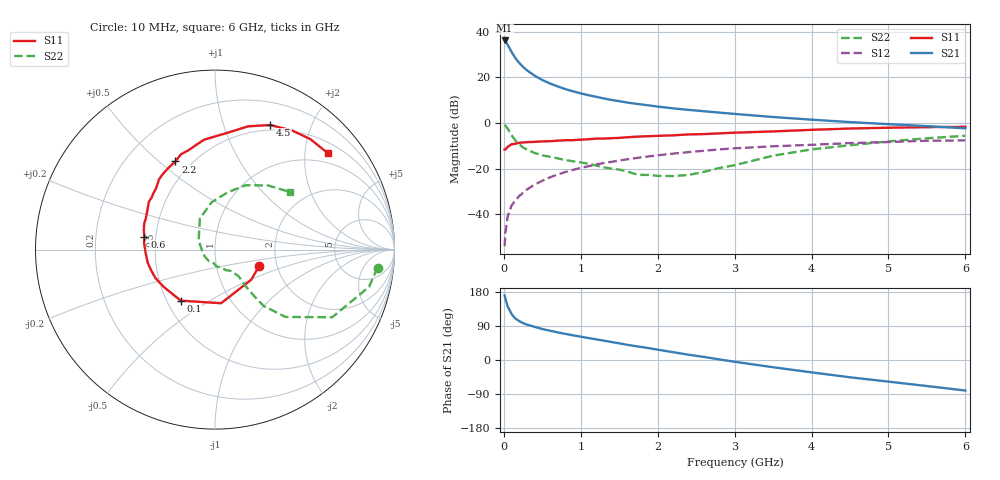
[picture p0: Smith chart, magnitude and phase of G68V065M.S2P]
! SIEMENS Small Signal Semiconductors
! BFG193
! Si NPN RF Bipolar Junction Transistor in SOT223
! VCE = 8 V  IC = 65 mA
! Common Emitter S-Parameters:  August  1996
# GHz  S  MA  R  50
!  f  S11  S21  S12  S22
! GHz  MAG  ANG  MAG  ANG  MAG  ANG  MAG  ANG
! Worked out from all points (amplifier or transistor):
!   36 points, 10 MHz to 6 GHz, reference 50 ohm
!   highest |S21| = 36.2 dB at 10 MHz (marker M1)
!   |S21| within 3 dB of that: start of sweep to 67.71 MHz
!   unconditionally stable (mu >= 1): 431.1 MHz to 2.36 GHz
!   at 250 MHz: K = 0.93, MSG = 27.6 dB, |S12| = -30.5 dB
!   at 1.4 GHz: K = 1.05, MAG = 12.3 dB, |S12| = -17.0 dB
!   at 6 GHz: K = 0.89, MSG = 2.7 dB, |S12| = -7.6 dB
!   S11 on the Smith chart (normalised r, x): 10 MHz: 1.62, -0.31; 100 MHz: 0.59, -0.38; 600 MHz: 0.43, +0.07; 2.2 GHz: 0.41, +0.57; 4.5 GHz: 0.44, +1.44; 6 GHz: 0.74, +2.51
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0.01  0.2628 -20.0  64.75 170.4  0.002 84.1  0.9112 -6.3
0.02  0.2626 -39.7  62.49 162.6  0.0039 74.0  0.8829 -13.6
0.05  0.3007 -83.5  52.02 141.3  0.0091 69.7  0.754 -30.0
0.1  0.3424 -123.8  36.41 121.5  0.0155 66.1  0.5431 -43.7
0.15  0.3532 -143.8  26.54 109.3  0.0202 66.5  0.4148 -49.2
0.2  0.3682 -154.6  20.88 102.6  0.025 67.8  0.3433 -49.8
0.25  0.3749 -162.9  17.02 97.3  0.0297 68.6  0.2919 -50.0
0.3  0.3818 -168.9  14.37 93.4  0.035 70.0  0.2631 -50.0
0.4  0.3871 -177.4  10.95 87.5  0.0447 69.6  0.2207 -49.1
0.5  0.3968 174.7  8.789 81.8  0.0544 68.9  0.1962 -48.5
0.6  0.4002 169.5  7.379 77.3  0.0646 68.0  0.1818 -49.5
0.7  0.4114 164.6  6.357 72.9  0.0747 66.8  0.1683 -51.4
0.8  0.4205 159.7  5.554 68.9  0.0845 64.6  0.1544 -53.0
1.1  0.4424 147.7  4.082 58.0  0.1131 59.6  0.1281 -62.8
1.3  0.4566 140.8  3.466 51.0  0.1331 55.5  0.1071 -69.8
1.6  0.4881 130.7  2.826 40.2  0.1603 48.9  0.0874 -88.7
2.2  0.5385 114.2  2.1 20.7  0.2139 35.3  0.0689 -149.2
2.8  0.5946 99.7  1.696 1.6  0.2643 21.4  0.1034 151.5
3.5  0.656 83.6  1.358 -19.1  0.3093 4.2  0.1927 115.9
4.5  0.7591 66.1  1.051 -45.6  0.3641 -15.9  0.3267 77.5
5.5  0.8133 49.1  0.857 -68.7  0.4102 -39.2  0.4634 50.5
6  0.8267 40.6  0.769 -80.6  0.4167 -52.6  0.5263 37.6
